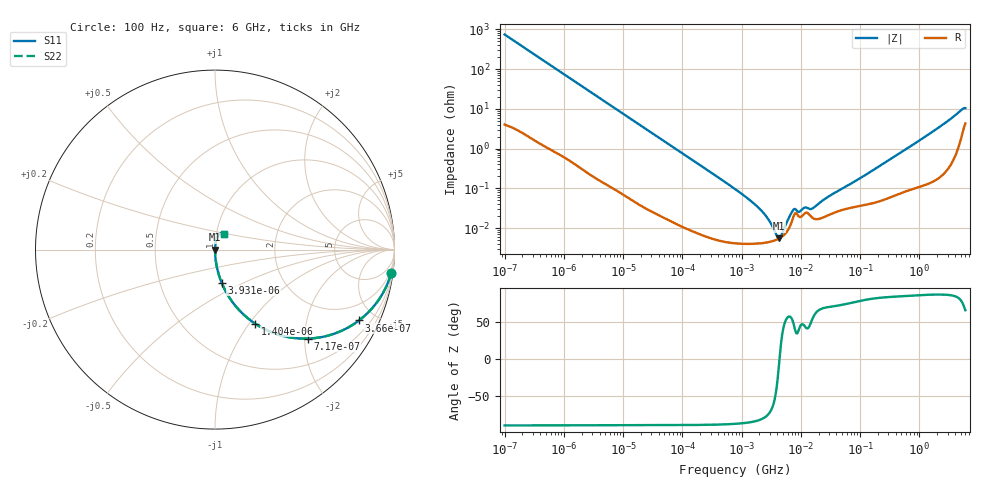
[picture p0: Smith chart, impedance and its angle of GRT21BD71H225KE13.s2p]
!Murata Part Number: GRT21BD71H225KE13
!These Parameters are Measured in Series Mode Connection
!Data Generated on Jun 19, 2026
!  o--ll--o
!Port1  Port2
!  o------o
!Operation Temp=25[degC], DC Bias Voltage=0[V]
!Freq. Start=100[Hz] Stop=6[GHz] 401[Steps]
# Hz S RI R 50
!Freq.(Hz) S11(Real) S11(Imag) S21(Real) S21(Imag) S12(Real) S12(Imag) S22(Real) S22(Imag)
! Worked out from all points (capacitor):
!   401 points, 100 Hz to 6 GHz, reference 50 ohm
!   read as one part in series: C = 2.15 uF near 109 Hz
!   lowest |Z| = 5.59 mohm at 4.246 MHz (marker M1)
!   series resonance near 4.366 MHz, so ESL is about 620 pH
!   S11 on the Smith chart (normalised r, x): 100 Hz: 1, -15; 366 Hz: 1.03, -4.05; 717 Hz: 1.02, -2.08; 1.404 kHz: 1.01, -1.06; 3.931 kHz: 1.00, -0.38; 6 GHz: 1.09, +0.19
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100  0.9813 -0.1329  0.0187 0.1329  0.0187 0.1329  0.9813 -0.1329
205  0.9275 -0.256  0.0725 0.256  0.0725 0.256  0.9275 -0.256
366  0.8023 -0.3947  0.1977 0.3947  0.1977 0.3947  0.8023 -0.3947
717  0.5185 -0.4958  0.4815 0.4958  0.4815 0.4958  0.5185 -0.4958
1404  0.2228 -0.4119  0.7772 0.4119  0.7772 0.4119  0.2228 -0.4119
2008  0.1241 -0.3256  0.8759 0.3256  0.8759 0.3256  0.1241 -0.3256
3931  0.0367 -0.1838  0.9633 0.1838  0.9633 0.1838  0.0367 -0.1838
10527  0.00578 -0.0713  0.9942 0.0713  0.9942 0.0713  0.00578 -0.0713
40335  0.000566 -0.0188  0.9994 0.0188  0.9994 0.0188  0.000566 -0.0188
774597  4.28e-05 -0.000968  1 0.000968  1 0.000968  4.28e-05 -0.000968
1983483  4.16e-05 -0.000313  1 0.000313  1 0.000313  4.16e-05 -0.000313
3549919  4.9e-05 -7.67e-05  1 7.67e-05  1 7.67e-05  4.9e-05 -7.67e-05
4246196  5.49e-05 -1.04e-05  0.9999 1.04e-05  0.9999 1.04e-05  5.49e-05 -1.04e-05
5311619  7e-05 7.75e-05  0.9999 -7.75e-05  0.9999 -7.75e-05  7e-05 7.75e-05
6948629  0.00014 0.000201  0.9999 -0.000201  0.9999 -0.000201  0.00014 0.000201
7599586  0.000205 0.000217  0.9998 -0.000217  0.9998 -0.000217  0.000205 0.000217
9506416  0.000193 0.000174  0.9998 -0.000174  0.9998 -0.000174  0.000193 0.000174
1.189169e7  0.000243 0.000229  0.9998 -0.000229  0.9998 -0.000229  0.000243 0.000229
1.555665e7  0.000186 0.00025  0.9998 -0.00025  0.9998 -0.00025  0.000186 0.00025
2.911731e7  0.000213 0.000585  0.9998 -0.000585  0.9998 -0.000585  0.000213 0.000585
3.124326e8  0.00061 0.00522  0.9994 -0.00522  0.9994 -0.00522  0.00061 0.00522
6e9  0.049 0.0867  0.951 -0.0867  0.951 -0.0867  0.049 0.0867
